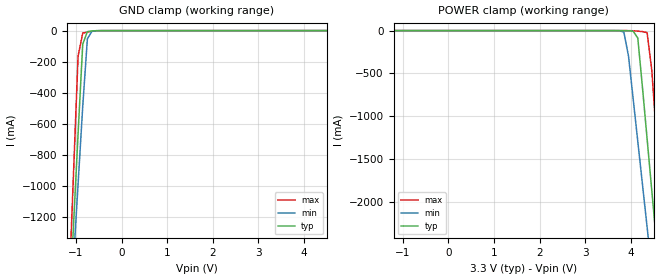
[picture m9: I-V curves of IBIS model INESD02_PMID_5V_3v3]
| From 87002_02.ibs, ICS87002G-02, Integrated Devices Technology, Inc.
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[Model] INESD02_PMID_5V_3v3
Model_type   Input
Polarity   Non-Inverting
Vinl = .8V
Vinh =  2V
|   typ   min   max
C_comp   2pF   1.5pF   2.5pF
|   typ   min   max
[Voltage range]  3.3V   3.15V   3.45V
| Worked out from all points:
|   GND clamp passes 1 mA (typ) near -0.58 V on its own axis
[GND_clamp]
|Voltage   I(typ)   I(min)   I(max)
-3.3V     -14.52A    -12.53A    -17.87A
-1.157V   -1.867A    -1.989A    -1.704A
-1.055V   -1.265A    -1.488A    -934.2mA
-952.6mV  -663.5mA   -987.5mA   -164.6mA
-850.5mV  -87.69mA   -487.6mA   -16.11mA
-748.5mV  -6.402mA   -52.83mA   -9.238mA
-646.4mV  -1.994mA   -2.763mA   -4.213mA
-340.2mV  -86.57uA   -101.8uA   -73.13uA
6.6V      207.5uA    263.8uA    158.1uA
[POWER_clamp]
|Voltage   I(typ)   I(min)   I(max)
-3.3V     207.5uA    255.1uA    163.5uA
3.64V     -86.57uA   -202uA     -61.97uA
3.844V    -498.9uA   -15.95mA   -88.54uA
3.946V    -1.994mA   -296.2mA   -353.3uA
4.048V    -6.402mA   -795.8mA   -1.999mA
4.151V    -87.69mA   -1.296A    -5.974mA
4.355V    -1.265A    -2.297A    -23.9mA
4.457V    -1.867A    -2.799A    -459.5mA
4.559V    -2.47A     -3.3A      -1.229A
4.661V    -3.072A    -3.801A    -1.999A
4.763V    -3.675A    -4.303A    -2.769A
6.6V      -14.52A    -13.34A    -16.63A
